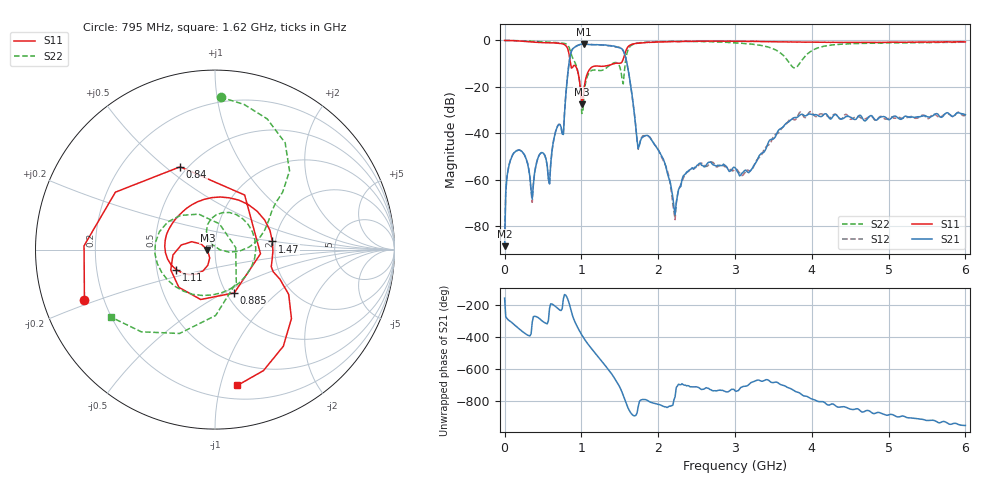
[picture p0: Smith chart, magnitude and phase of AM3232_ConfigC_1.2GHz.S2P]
! Network Analyzer HP8753E.07.74: Oct 30, 2002 Serial No. US37390186
! 24 Jul 2023  10:51:43
! Frequency  S11  S21  S12  S22
# HZ  S  DB R  50
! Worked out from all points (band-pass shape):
!   401 points, 30 kHz to 6 GHz, reference 50 ohm
!   highest |S21| = -1.53 dB at 1.035 GHz (marker M1); lowest = -88.5 dB at 30 kHz (marker M2)
!   |S21| within 3 dB of the highest: 870.8 MHz to 1.548 GHz (676.7 MHz wide, 56 % of centre)
!   lowest |S11| = -27.5 dB at 1.005 GHz (marker M3), VSWR 1.09, Z = 46 - j0.183 ohm
!   |S11| at or under -10 dB: 859.4 MHz to 1.422 GHz (562.3 MHz wide, 49.3 % of centre)
!   |S22| runs from -31.5 to 0.0 dB; largest |S21 - S12| = 0.04
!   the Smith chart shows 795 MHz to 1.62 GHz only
!   S11 on the Smith chart (normalised r, x): 795 MHz: 0.13, -0.18; 840 MHz: 0.46, +0.56; 885 MHz: 1.09, -0.56; 1.11 GHz: 0.63, -0.15; 1.47 GHz: 1.93, +0.20; 1.62 GHz: 0.31, -1.13
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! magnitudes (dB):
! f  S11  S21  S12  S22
! 30 kHz  0.0  -88.5  -84.8  0.0
! 135 MHz  -0.1  -48.0  -47.8  -0.1
! 360 MHz  -0.6  -68.2  -69.7  -0.3
! 465 MHz  -0.9  -48.6  -48.7  -0.5
! 585 MHz  -1.0  -61.8  -62.1  -0.7
! 795 MHz  -2.2  -24.4  -24.0  -1.4
! 840 MHz  -6.0  -9.5  -9.4  -3.0
! 885 MHz  -11.6  -3.6  -3.7  -7.5
! 1.005 GHz  -27.5  -1.6  -1.6  -31.5
! 1.035 GHz  -20.4  -1.5  -1.6  -22.8
! 1.11 GHz  -12.3  -1.8  -1.7  -13.6
! 1.47 GHz  -9.8  -2.9  -2.8  -9.7
! 1.62 GHz  -2.3  -14.7  -14.8  -3.2
! 1.74 GHz  -1.2  -46.5  -46.8  -1.1
! 2.01 GHz  -0.6  -47.7  -47.5  -0.5
! 2.22 GHz  -0.5  -74.9  -77.1  -0.4
! 2.415 GHz  -0.4  -55.6  -55.5  -0.4
! 3 GHz  -0.3  -54.8  -55.5  -1.0
! 3.78 GHz  -0.7  -33.1  -34.2  -11.8
! 4.005 GHz  -0.7  -31.9  -31.1  -4.3
! 5.01 GHz  -0.8  -34.1  -33.3  -1.0
! 6 GHz  -0.6  -31.9  -32.0  -0.7
